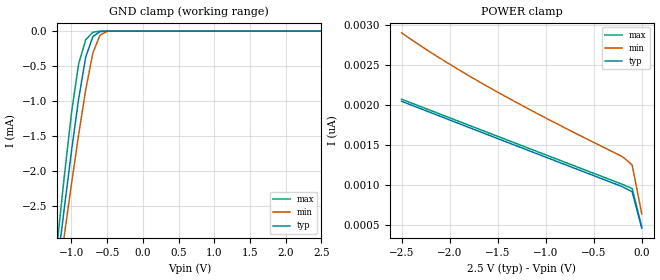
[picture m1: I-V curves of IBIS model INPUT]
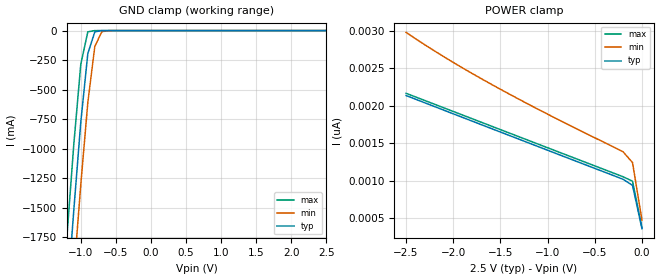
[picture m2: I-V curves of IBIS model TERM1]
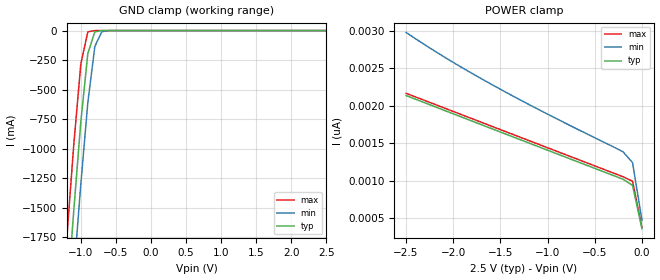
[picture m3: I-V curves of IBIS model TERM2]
|   PERICOM SEMICONDUCTOR CORP
|   IBIS Model of PI3CH480
|   Product Family: 3CH
|   TSSOP (L) Package
[IBIS Ver] 3.2
[Comment char] |_char
[File Name] pi3ch480_l_25v.ibs
[File Rev] 1.0
[Source] File originated at Pericom Semiconductor Corp.
[Date] 11/20/15
[Disclaimer] (C) Copyright PERICOM Semiconductor Corporation
   All rights reserved
  Pericom Semiconductor Corporation hereby grants the user of
  this IBIS model a non-exclusive, nontransferable license to
  use this IBIS model under the following terms.
  This IBIS model is provided on an "AS IS" basis and Pericom
  makes absolutely no warranty with respect to the information
  contained herein. PERICOM DISCLAIMS AND CUSTOMER WAIVES ALL
  WARRANTIES, EXPRESSED OR IMPLIED, INCLUDING WARRANTIES OF
  MERCHANTABILITY OR FITNESS FOR A PARTICULAR PURPOSE. The
  entire risk as to quality and performance is with the customer.
  Accordingly, in no event shall the company be liable for any
  damages, whether in contract or tort, including any lost
  profits or other incidental, consequential, exemplary, or
  punitive damages arising out of the use or application of the
  IBIS model provided in this package. Further, Pericom reserves
  the right to make changes without notice to any product herein
  to improve reliability, function, or design. Pericom does not
  convey any license under patent rights or any other intellectual
  property rights, including those of third parties.
  The user is granted this license only to use the IBIS model
  and is not granted rights to sell, load, rent, lease or license
  the IBIS model in whole or in part, or in modified form to anyone
  other than user. User may modify the IBIS model to suit its specific
  application but rights to derivative works and such modifications
  shall belong to Pericom.
  Pericom is not obligated to provide maintenance or support
  for the licensed IBIS model.
  Contact Pericom at ATTN: APPLICATION ENGINEERING / IBIS MODELS
  1545 Barber Lane Milpitas, CA 95035 USA.
[Component] PI3CH480
[Manufacturer] Pericom Semiconductor Corp.
[Package]
| variable   typ   min   max
R_pkg   0.05122ohm   0.05070ohm   0.05174ohm
L_pkg   2.82616nH   2.45517nH   3.19714nH
C_pkg   0.42513pF   0.33872pF   0.51154pF
[Pin]   signal_name   model_name   R_pin   L_pin   C_pin
1   S   INPUT   0.05174   3.19714nH   0.51154pF
2   IA0   TERM1   0.05140   2.94981nH   0.45394pF
3   IA1   TERM1   0.05105   2.70250nH   0.39633pF
4   YA   TERM2   0.05070   2.45517nH   0.33872pF
5   IB0   TERM1   0.05070   2.45517nH   0.33872pF
6   IB1   TERM1   0.05105   2.70250nH   0.39633pF
7   YB   TERM2   0.05140   2.94981nH   0.45394pF
8   GND   GND   0.05174   3.19714nH   0.51154pF
9   YC   TERM2   0.05174   3.19714nH   0.51154pF
10   IC1   TERM1   0.05140   2.94981nH   0.45394pF
11   IC0   TERM1   0.05105   2.70250nH   0.39633pF
12   YD   TERM2   0.05070   2.45517nH   0.33872pF
13   ID1   TERM1   0.05070   2.45517nH   0.33872pF
14   ID0   TERM1   0.05105   2.70250nH   0.39633pF
15   _EN   INPUT   0.05140   2.94981nH   0.45394pF
16   VCC   POWER   0.05174   3.19714nH   0.51154pF
[Series Switch Groups]
On 1 /
Off 2 /
[Series Pin Mapping]   pin_2   model_name  function_table_group
2   4   SWITCH1   1
5   7   SWITCH1   1
11   9   SWITCH1   1
14   12   SWITCH1   1
3   4   SWITCH1   2
6   7   SWITCH1   2
10   9   SWITCH1   2
13   12   SWITCH1   2
|   Model SWITCH1
[Model] SWITCH1
Model_type Series_switch
| variable   typ   min   max
C_comp   6.40pF   6.30pF   6.50pF
[Voltage Range]   2.500V   2.250V   2.750V
[GND Clamp Reference]   0.000V   0.000V   0.000V
[POWER Clamp Reference]   2.500V   2.250V   2.750V
[On]
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[OFF]
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| Models and submodels in the file (4): INPUT (Input), SWITCH1 (Series_switch), TERM1 (Terminator), TERM2 (Terminator)
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|   Model INPUT
[Model] INPUT
Model_type Input
Vinl = 0.800V
Vinh = 1.800V
| variable   typ   min   max
C_comp   1.800pF   1.700pF   1.900pF
[Voltage Range]   2.500V   2.250V   2.750V
[GND Clamp Reference]   0.000V   0.000V   0.000V
[POWER Clamp Reference]   2.500V   2.250V   2.750V
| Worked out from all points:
|   GND clamp passes 1 mA (typ) near -0.90 V on its own axis
[GND Clamp]
| Voltage   I(typ)   I(min)   I(max)
-2.5V     -14.74mA   -13.73mA   -16.44mA
-1.2V     -3.364mA   -3.668mA   -3.042mA
-1.1V     -2.528mA   -2.921mA   -2.075mA
-1V       -1.72mA    -2.189mA   -1.175mA
-900mV    -970.6uA   -1.485mA   -470.9uA
-800mV    -370.2uA   -835.9uA   -124.8uA
-700mV    -77.27uA   -313.6uA   -15.69uA
-600mV    -8.132uA   -56.97uA   -899.1nA
-500mV    -581.9nA   -5.514uA   -27.41nA
2.5V      456.5pA    1.382nA    21.38pA
[POWER Clamp]   |Note: Vtable = Vcc - Voutput
| Voltage   I(typ)   I(min)   I(max)
-2.5V     2.046nA    2.904nA    2.072nA
-2.1V     1.859nA    2.586nA    1.886nA
-1.6V     1.626nA    2.228nA    1.654nA
-1V       1.347nA    1.838nA    1.376nA
-200mV    975.5pA    1.351nA    1.005nA
-100mV    912.5pA    1.249nA    952.9pA
0V        456.5pA    636.6pA    471.6pA
|   Model TERM1
[Model] TERM1
Model_type Terminator
| variable   typ   min   max
C_comp   3.200pF   3.150pF   3.350pF
[Voltage Range]   2.500V   2.250V   2.750V
[GND Clamp Reference]   0.000V   0.000V   0.000V
[POWER Clamp Reference]   2.500V   2.250V   2.750V
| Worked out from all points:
|   GND clamp passes 1 mA (typ) near -0.71 V on its own axis
[GND Clamp]
| Voltage   I(typ)   I(min)   I(max)
-2.5V     -12.6A     -12.86A    -12.34A
-1.2V     -2.312A    -2.839A    -1.76A
-1.1V     -1.522A    -2.068A    -964.6mA
-1V       -774.2mA   -1.302A    -284.3mA
-900mV    -194.8mA   -609.8mA   -10.79mA
-800mV    -10.29mA   -134.3mA   -176uA
-700mV    -369.5uA   -9.267mA   -1.644uA
-500mV    -244.1nA   -27.85uA   -129.7pA
2.5V      361.1pA    1.419nA    73.2pA
[POWER Clamp]   |Note: Vtable = Vcc - Voutput
| Voltage   I(typ)   I(min)   I(max)
-2.5V     2.136nA    2.978nA    2.166nA
-2.1V     1.941nA    2.654nA    1.972nA
-1.6V     1.698nA    2.289nA    1.73nA
-1V       1.407nA    1.888nA    1.44nA
-200mV    1.019nA    1.386nA    1.053nA
-100mV    938.7pA    1.242nA    993.5pA
0V        361.1pA    474.5pA    376.7pA
|   Model TERM2
[Model] TERM2
Model_type Terminator
| variable   typ   min   max
C_comp   3.200pF   3.150pF   3.350pF
[Voltage Range]   2.500V   2.250V   2.750V
[GND Clamp Reference]   0.000V   0.000V   0.000V
[POWER Clamp Reference]   2.500V   2.250V   2.750V
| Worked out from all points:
|   GND clamp passes 1 mA (typ) near -0.71 V on its own axis
[GND Clamp]
| Voltage   I(typ)   I(min)   I(max)
-2.5V     -12.6A     -12.86A    -12.34A
-1.2V     -2.312A    -2.839A    -1.76A
-1.1V     -1.522A    -2.068A    -964.6mA
-1V       -774.2mA   -1.302A    -284.3mA
-900mV    -194.8mA   -609.8mA   -10.79mA
-800mV    -10.29mA   -134.3mA   -176uA
-700mV    -369.5uA   -9.267mA   -1.644uA
-500mV    -244.1nA   -27.85uA   -129.7pA
2.5V      361.1pA    1.419nA    73.2pA
[POWER Clamp]   |Note: Vtable = Vcc - Voutput
| Voltage   I(typ)   I(min)   I(max)
-2.5V     2.136nA    2.978nA    2.166nA
-2.1V     1.941nA    2.654nA    1.972nA
-1.6V     1.698nA    2.289nA    1.73nA
-1V       1.407nA    1.888nA    1.44nA
-200mV    1.019nA    1.386nA    1.053nA
-100mV    938.7pA    1.242nA    993.5pA
0V        361.1pA    474.6pA    376.7pA
